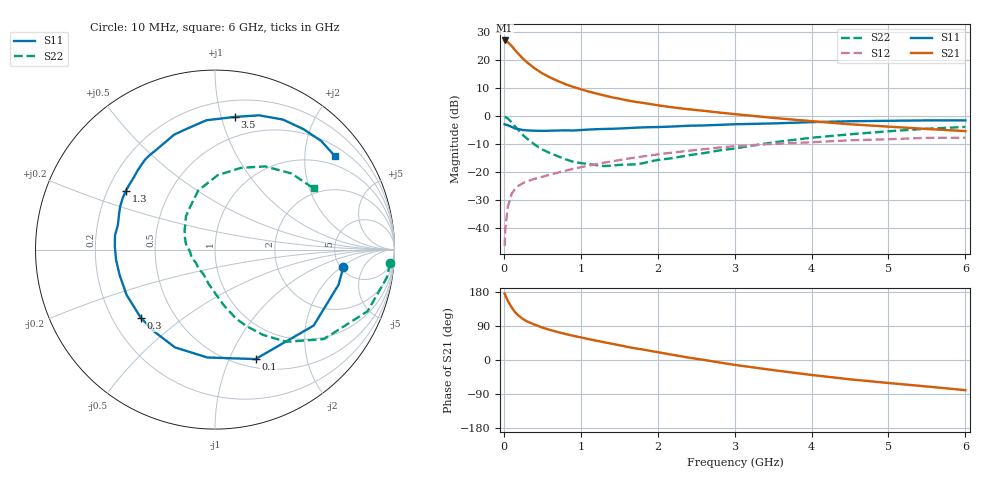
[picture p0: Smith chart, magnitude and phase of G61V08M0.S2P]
! SIEMENS Small Signal Semiconductors
! BFG193
! Si NPN RF Bipolar Junction Transistor in SOT223
! VCE = 1 V  IC = 8 mA
! Common Emitter S-Parameters:  August  1996
# GHz  S  MA  R  50
!  f  S11  S21  S12  S22
! GHz  MAG  ANG  MAG  ANG  MAG  ANG  MAG  ANG
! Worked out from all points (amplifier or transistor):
!   36 points, 10 MHz to 6 GHz, reference 50 ohm
!   highest |S21| = 27.1 dB at 10 MHz (marker M1)
!   |S21| within 3 dB of that: start of sweep to 132.4 MHz
!   unconditionally stable (mu >= 1): 883.4 MHz to 2.976 GHz
!   at 250 MHz: K = 0.48, MSG = 22.2 dB, |S12| = -23.8 dB
!   at 1.4 GHz: K = 1.09, MAG = 9.7 dB, |S12| = -16.1 dB
!   at 6 GHz: K = 0.96, MSG = 1.2 dB, |S12| = -7.6 dB
!   S11 on the Smith chart (normalised r, x): 10 MHz: 5.25, -2.17; 100 MHz: 0.59, -1.26; 300 MHz: 0.32, -0.35; 1.3 GHz: 0.28, +0.28; 3.5 GHz: 0.33, +1.10; 6 GHz: 0.74, +2.73
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0.01  0.7215 -7.9  22.66 175.1  0.0048 87.7  0.9787 -4.5
0.02  0.7156 -15.9  22.43 171.0  0.01 83.2  0.97 -9.2
0.05  0.6938 -37.6  21.26 156.5  0.0237 72.5  0.9169 -22.0
0.1  0.6504 -69.7  18.21 139.4  0.0412 59.8  0.7853 -39.4
0.15  0.6025 -94.1  14.97 125.0  0.0518 50.6  0.6501 -52.2
0.2  0.5887 -112.3  12.63 115.7  0.0588 46.9  0.5469 -60.5
0.25  0.5686 -126.4  10.7 108.0  0.0644 43.7  0.4603 -67.7
0.3  0.5616 -137.4  9.227 102.1  0.0688 42.3  0.4021 -73.0
0.4  0.5534 -153.0  7.21 93.3  0.0764 41.3  0.3132 -81.1
0.5  0.5501 -165.2  5.858 85.6  0.0832 40.9  0.2558 -87.8
0.6  0.5541 -174.1  4.955 79.5  0.0909 41.5  0.2202 -93.9
0.8  0.5628 171.9  3.757 68.7  0.1065 41.5  0.1714 -107.1
0.9  0.5581 165.9  3.361 64.0  0.1155 41.3  0.1546 -113.3
1.1  0.5805 155.6  2.777 55.3  0.1314 40.6  0.1408 -128.6
1.3  0.5949 146.7  2.367 46.9  0.1487 38.7  0.1294 -144.6
1.7  0.6252 131.1  1.825 31.1  0.1829 33.5  0.1385 -173.7
2.2  0.6583 115.2  1.442 13.5  0.2262 24.5  0.18 158.6
2.8  0.7038 98.6  1.17 -6.4  0.2773 12.4  0.2462 131.1
3.5  0.7473 81.6  0.939 -26.6  0.3217 -3.9  0.3425 105.8
4.5  0.8175 62.4  0.722 -51.0  0.3735 -23.0  0.4779 72.4
5.5  0.8464 45.7  0.595 -69.9  0.4132 -45.8  0.6009 44.9
6  0.8472 37.9  0.545 -79.6  0.4148 -58.9  0.6472 31.8
